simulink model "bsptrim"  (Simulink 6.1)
settings: Solver=ode45  StartTime=0.0  StopTime=100  RelTol=1e-3

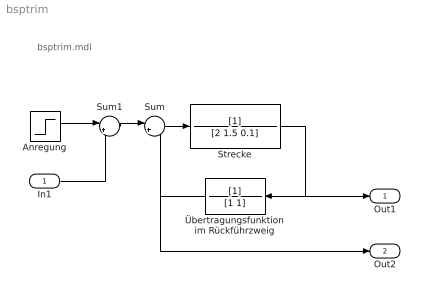
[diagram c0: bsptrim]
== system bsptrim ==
  note: bsptrim.mdl
  In1 : Inport  Port=1  LatchInput=off
  Anregung : Step  SampleTime=0
  Strecke : TransferFcn  Denominator=[2 1.5 0.1]
  Sum : Sum  Inputs=|+-
  Sum1 : Sum  Inputs=|++
  Übertragungsfunktion im Rückführzweig : TransferFcn  Orientation=left  Denominator=[1 1]
  Out1 : Outport
  Out2 : Outport  Port=2
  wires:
  Sum/1 -> Strecke/1
  Sum1/1 -> Sum/1
  Anregung/1 -> Sum1/1
  In1/1 -> Sum1/2
  Übertragungsfunktion im Rückführzweig/1 -> Sum/2, Out2/1
  Strecke/1 -> Übertragungsfunktion im Rückführzweig/1, Out1/1
